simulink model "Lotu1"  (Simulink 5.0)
settings: Solver=ode45  StartTime=0.0  StopTime=10.0  RelTol=1e-3

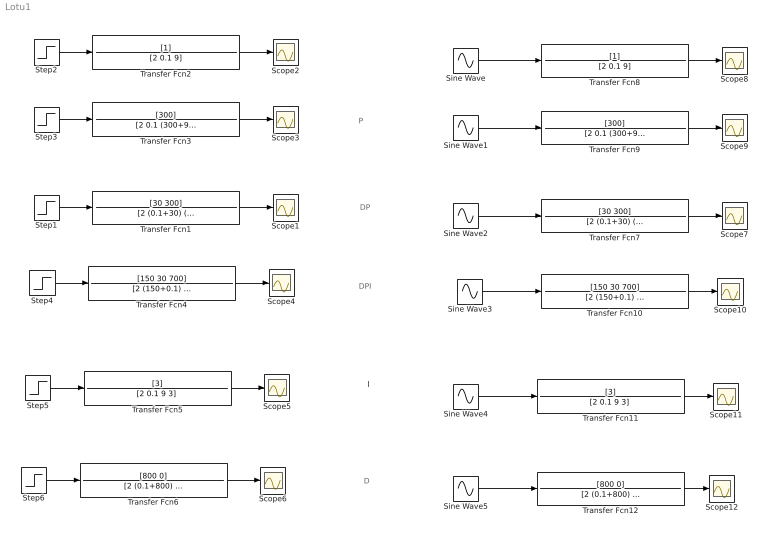
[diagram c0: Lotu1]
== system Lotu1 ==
  note: P
  note: DP
  note: DPI
  note: I
  note: D
  Scope{1..12} (12 alike) : Scope
  Sine Wave{,1..5} (6 alike) : Sin  SampleTime=0
  Step{1..6} (6 alike) : Step  Time=0  SampleTime=0
  Transfer Fcn1 : TransferFcn  Numerator=[30 300]  Denominator=[2 (0.1+30) (300+9)]
  Transfer Fcn10 : TransferFcn  Numerator=[150 30 700]  Denominator="[2 (150+0.1)  (30+9) 700]"
  Transfer Fcn11 : TransferFcn  Numerator=[3]  Denominator=[2 0.1 9 3]
  Transfer Fcn12 : TransferFcn  Numerator=[800 0]  Denominator=[2 (0.1+800) 9]
  Transfer Fcn2 : TransferFcn  Denominator=[2 0.1 9]
  Transfer Fcn3 : TransferFcn  Numerator=[300]  Denominator=[2 0.1 (300+9)]
  Transfer Fcn4 : TransferFcn  Numerator=[150 30 700]  Denominator="[2 (150+0.1)  (30+9) 700]"
  Transfer Fcn5 : TransferFcn  Numerator=[3]  Denominator=[2 0.1 9 3]
  Transfer Fcn6 : TransferFcn  Numerator=[800 0]  Denominator=[2 (0.1+800) 9]
  Transfer Fcn7 : TransferFcn  Numerator=[30 300]  Denominator=[2 (0.1+30) (300+9)]
  Transfer Fcn8 : TransferFcn  Denominator=[2 0.1 9]
  Transfer Fcn9 : TransferFcn  Numerator=[300]  Denominator=[2 0.1 (300+9)]
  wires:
  Step2/1 -> Transfer Fcn2/1
  Transfer Fcn2/1 -> Scope2/1
  Step3/1 -> Transfer Fcn3/1
  Transfer Fcn3/1 -> Scope3/1
  Step1/1 -> Transfer Fcn1/1
  Step4/1 -> Transfer Fcn4/1
  Transfer Fcn4/1 -> Scope4/1
  Transfer Fcn1/1 -> Scope1/1
  Step5/1 -> Transfer Fcn5/1
  Transfer Fcn5/1 -> Scope5/1
  Step6/1 -> Transfer Fcn6/1
  Transfer Fcn6/1 -> Scope6/1
  Transfer Fcn8/1 -> Scope8/1
  Transfer Fcn9/1 -> Scope9/1
  Transfer Fcn10/1 -> Scope10/1
  Transfer Fcn7/1 -> Scope7/1
  Transfer Fcn11/1 -> Scope11/1
  Transfer Fcn12/1 -> Scope12/1
  Sine Wave/1 -> Transfer Fcn8/1
  Sine Wave1/1 -> Transfer Fcn9/1
  Sine Wave2/1 -> Transfer Fcn7/1
  Sine Wave3/1 -> Transfer Fcn10/1
  Sine Wave4/1 -> Transfer Fcn11/1
  Sine Wave5/1 -> Transfer Fcn12/1
